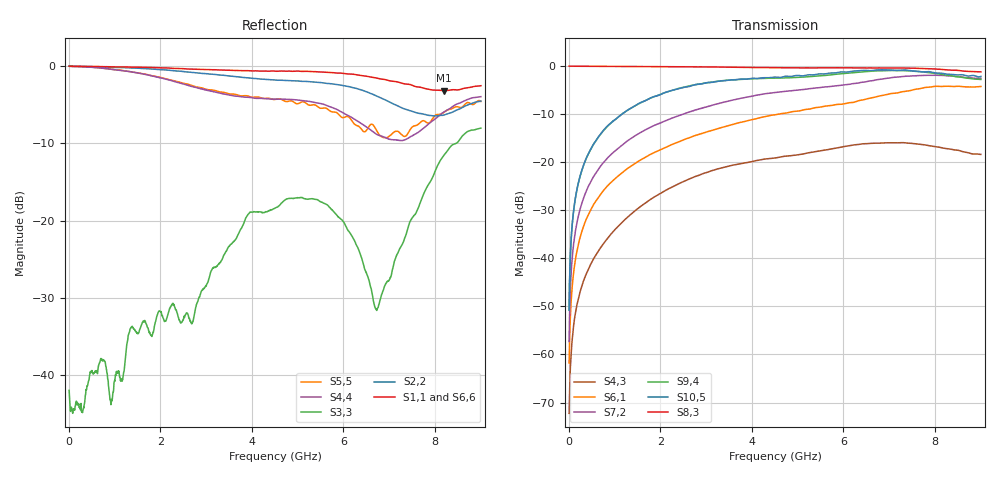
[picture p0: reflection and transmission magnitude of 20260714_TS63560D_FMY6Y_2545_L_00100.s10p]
# GHz S DB R 50
! CMT, SN0916, 25263762, 26.7.0
! Date: 15.07.2026 13:34:04
! Data: Format
! Freq S1.1:dB/Ang S1.2:dB/Ang S1.3:dB/Ang S1.4:dB/Ang S1.5:dB/Ang S1.6:dB/Ang S1.7:dB/Ang S1.8:dB/Ang S1.9:dB/Ang S1.10:dB/Ang
!  S2.1:dB/Ang S2.2:dB/Ang S2.3:dB/Ang S2.4:dB/Ang S2.5:dB/Ang S2.6:dB/Ang S2.7:dB/Ang S2.8:dB/Ang S2.9:dB/Ang S2.10:dB/Ang
!  S3.1:dB/Ang S3.2:dB/Ang S3.3:dB/Ang S3.4:dB/Ang S3.5:dB/Ang S3.6:dB/Ang S3.7:dB/Ang S3.8:dB/Ang S3.9:dB/Ang S3.10:dB/Ang
!  S4.1:dB/Ang S4.2:dB/Ang S4.3:dB/Ang S4.4:dB/Ang S4.5:dB/Ang S4.6:dB/Ang S4.7:dB/Ang S4.8:dB/Ang S4.9:dB/Ang S4.10:dB/Ang
!  S5.1:dB/Ang S5.2:dB/Ang S5.3:dB/Ang S5.4:dB/Ang S5.5:dB/Ang S5.6:dB/Ang S5.7:dB/Ang S5.8:dB/Ang S5.9:dB/Ang S5.10:dB/Ang
!  S6.1:dB/Ang S6.2:dB/Ang S6.3:dB/Ang S6.4:dB/Ang S6.5:dB/Ang S6.6:dB/Ang S6.7:dB/Ang S6.8:dB/Ang S6.9:dB/Ang S6.10:dB/Ang
!  S7.1:dB/Ang S7.2:dB/Ang S7.3:dB/Ang S7.4:dB/Ang S7.5:dB/Ang S7.6:dB/Ang S7.7:dB/Ang S7.8:dB/Ang S7.9:dB/Ang S7.10:dB/Ang
!  S8.1:dB/Ang S8.2:dB/Ang S8.3:dB/Ang S8.4:dB/Ang S8.5:dB/Ang S8.6:dB/Ang S8.7:dB/Ang S8.8:dB/Ang S8.9:dB/Ang S8.10:dB/Ang
!  S9.1:dB/Ang S9.2:dB/Ang S9.3:dB/Ang S9.4:dB/Ang S9.5:dB/Ang S9.6:dB/Ang S9.7:dB/Ang S9.8:dB/Ang S9.9:dB/Ang S9.10:dB/Ang
!  S10.1:dB/Ang S10.2:dB/Ang S10.3:dB/Ang S10.4:dB/Ang S10.5:dB/Ang S10.6:dB/Ang S10.7:dB/Ang S10.8:dB/Ang S10.9:dB/Ang S10.10:dB/Ang
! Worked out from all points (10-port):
!   2001 points, 10 MHz to 9 GHz, reference 50 ohm
!   strongest paths, dB at 10 MHz, 2.257 GHz, 4.505 GHz, 6.753 GHz, 9 GHz:
!     S8,3: -0.1, -0.2, -0.4, -0.4, -1.3
!     S10,5: -50.8, -5.1, -2.3, -0.8, -2.2
!     S9,4: -50.8, -5.1, -2.6, -1.0, -2.8
!     S7,2: -57.3, -10.9, -5.5, -2.9, -2.6
!     S6,1: -61.8, -16.4, -10.2, -6.3, -4.3
!     S4,3: -72.2, -25.2, -19.2, -16.1, -18.4
!   lowest |S11| = -3.2 dB at 8.2 GHz (marker M1), VSWR 5.55, Z = 11.1 - j23.7 ohm
!   |S11| at or under -10 dB: nowhere
